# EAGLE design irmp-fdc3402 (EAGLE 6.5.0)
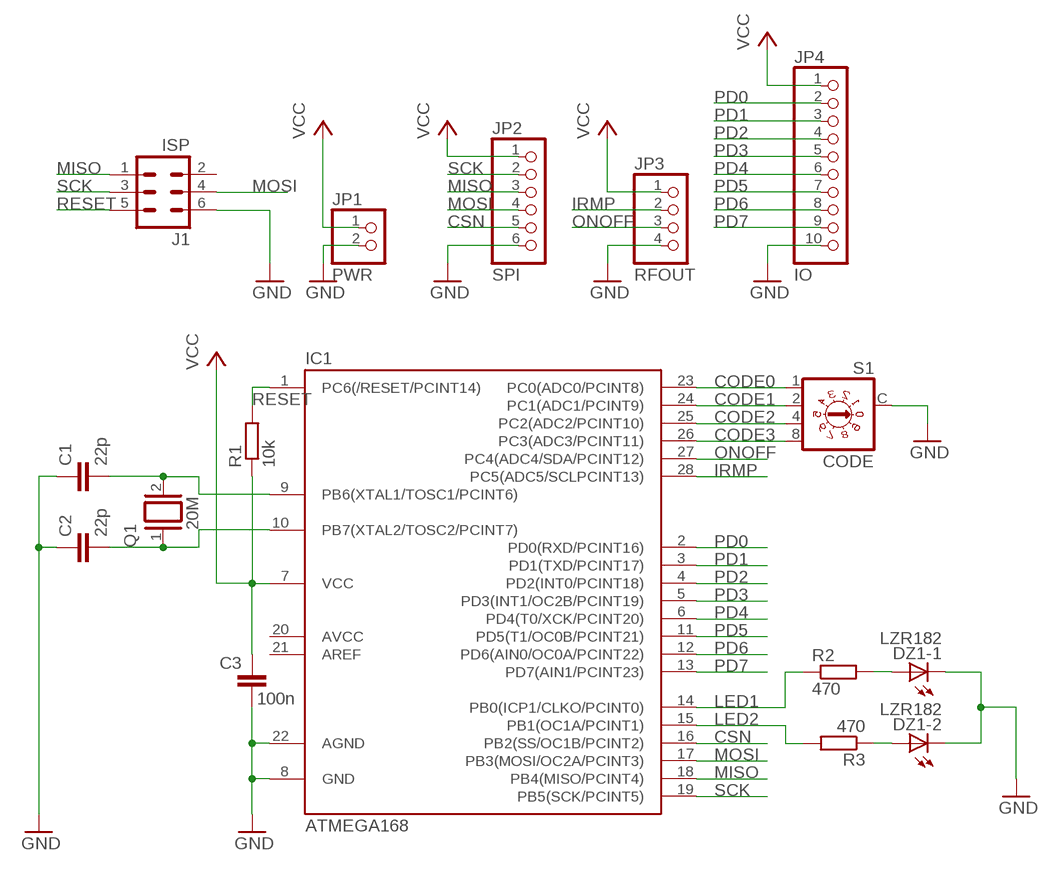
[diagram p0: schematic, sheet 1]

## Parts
C1  22p  C-EU025-024X044  [C025-024X044]
C2  22p  C-EU025-024X044  [C025-024X044]
C3  100n  C-EU025-024X044  [C025-024X044]
DZ1  LZR182  [LZR182]
IC1  ATMEGA168  MEGA48/88/168-PU  [DIL28-3]
J1  ISP  ML6  [ML6]
JP1  PWR  PINHD-1X2  [1X02]
JP2  SPI  PINHD-1X6  [1X06]
JP3  RFOUT  PINHD-1X4  [1X04]
JP4  IO  PINHD-1X10  [1X10]
Q1  20M  XTAL/S  [QS]
R1  10k  R-EU_0207/10  [0207/10]
R2  470  R-EU_0207/10  [0207/10]
R3  470  R-EU_0207/10  [0207/10]
S1  CODE  DRS3010  [DRR3010]

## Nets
CODE0: IC1.23(PC0(ADC0/PCINT8)) S1.1
CODE1: IC1.24(PC1(ADC1/PCINT9)) S1.2
CODE2: IC1.25(PC2(ADC2/PCINT10)) S1.4
CODE3: IC1.26(PC3(ADC3/PCINT11)) S1.8
CSN: IC1.16(PB2(SS/OC1B/PCINT2)) JP2.5
GND: C1.1 C2.1 C3.1 DZ1.K1(-1:C) DZ1.K2(-2:C) IC1.8(GND) IC1.22(AGND) J1.6 JP1.2 JP2.6 JP3.4 JP4.10 S1.C
IRMP: IC1.28(PC5(ADC5/SCLPCINT13)) JP3.2
LED1: IC1.14(PB0(ICP1/CLKO/PCINT0)) R2.1
LED2: IC1.15(PB1(OC1A/PCINT1)) R3.2
MISO: IC1.18(PB4(MISO/PCINT4)) J1.1 JP2.3
MOSI: IC1.17(PB3(MOSI/OC2A/PCINT3)) J1.4 JP2.4
N$1: DZ1.A1(-1:A) R2.2
N$2: DZ1.A2(-2:A) R3.1
ONOFF: IC1.27(PC4(ADC4/SDA/PCINT12)) JP3.3
PD0: IC1.2(PD0(RXD/PCINT16)) JP4.2
PD1: IC1.3(PD1(TXD/PCINT17)) JP4.3
PD2: IC1.4(PD2(INT0/PCINT18)) JP4.4
PD3: IC1.5(PD3(INT1/OC2B/PCINT19)) JP4.5
PD4: IC1.6(PD4(T0/XCK/PCINT20)) JP4.6
PD5: IC1.11(PD5(T1/OC0B/PCINT21)) JP4.7
PD6: IC1.12(PD6(AIN0/OC0A/PCINT22)) JP4.8
PD7: IC1.13(PD7(AIN1/PCINT23)) JP4.9
RESET: IC1.1(PC6(/RESET/PCINT14)) J1.5 R1.2
SCK: IC1.19(PB5(SCK/PCINT5)) J1.3 JP2.2
VCC: C3.2 IC1.7(VCC) JP1.1 JP2.1 JP3.1 JP4.1 R1.1
XTAL1: C1.2 IC1.9(PB6(XTAL1/TOSC1/PCINT6)) Q1.2
XTAL2: C2.2 IC1.10(PB7(XTAL2/TOSC2/PCINT7)) Q1.1
Unconnected: IC1.20(AVCC) IC1.21(AREF) J1.2

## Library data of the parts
C1-C3 = rcl:C-EU: CAPACITOR, European symbol
DZ1 = led:LZR182: LED BLOCK 2 LEDs, Siemens
IC1 = avr-7:MEGA48/88/168-PU
J1 = con-harting-ml:ML6: HARTING; OC_FARNELL: unknown; OC_NEWARK: unknown
JP1 = pinhead:PINHD-1X2: PIN HEADER
JP2 = pinhead:PINHD-1X6: PIN HEADER
JP3 = pinhead:PINHD-1X4: PIN HEADER
JP4 = pinhead:PINHD-1X10: PIN HEADER
Q1 = special:XTAL/S: CRYSTAL
R1-R3 = rcl:R-EU_: RESISTOR, European symbol
S1 = switch-dil:DRS3010: DIL/CODE SWITCH; MPN: DRS3010; OC_FARNELL: 1190426; OC_NEWARK: 01M7366

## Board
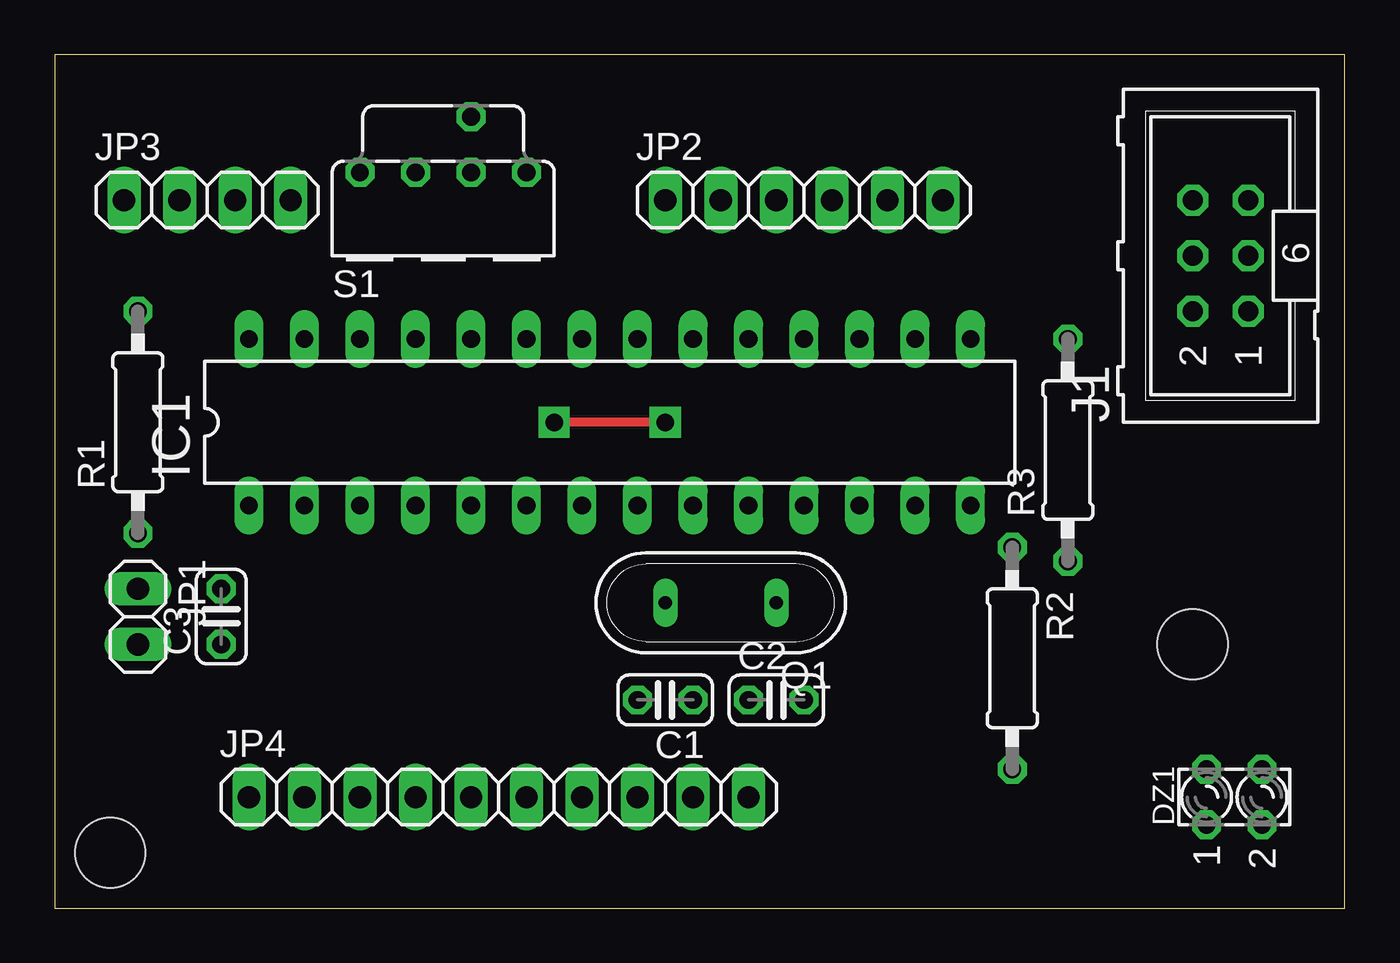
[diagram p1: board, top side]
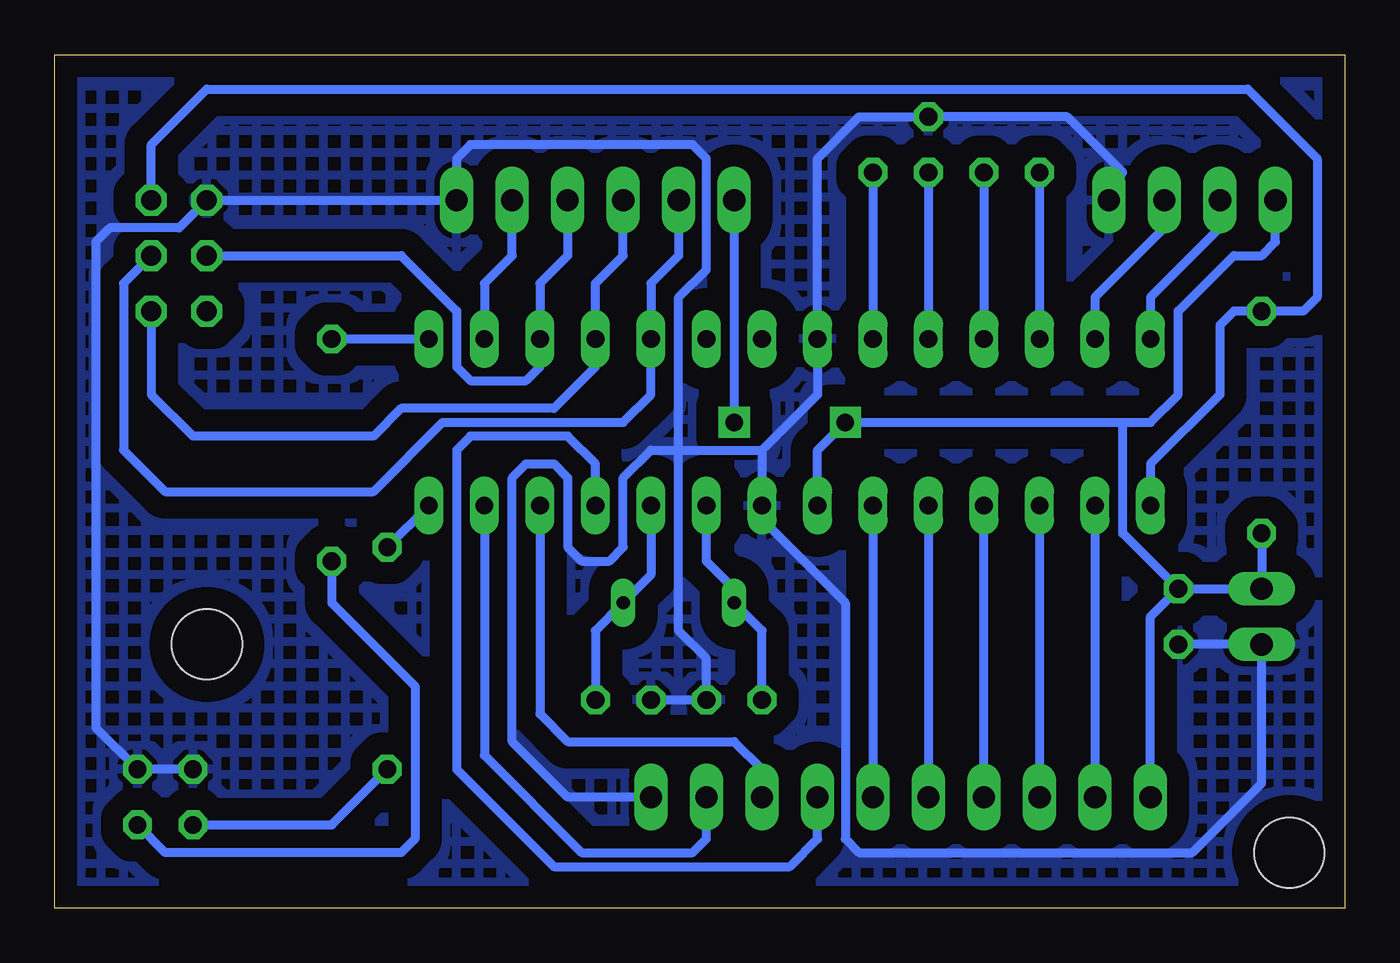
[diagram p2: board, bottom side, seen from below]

Size 59.03 x 39.04 mm. Coordinates in mm from the lower left corner, seen from the top.
Outline: 0,0 59.03,0 59.03,39.04 0,39.04 0,0
Copper layers (1*16): Top 0.035mm / dielectric 1.5mm / Bottom 0.035mm
Design rules "default": minimum track width 10mil, minimum drill 24mil, track to track 8mil, track to pad 8mil, pad to pad 8mil, via to via 8mil, smd to smd 8mil, copper to edge 40mil, drill to drill 8mil, minimum pad ring 10mil, minimum via ring 8mil, stop-mask expansion 4mil, vias tented up to drill 0mil, thermal gap 10mil
Holes 3.2 mm at 2.54,2.54 52.07,12.06

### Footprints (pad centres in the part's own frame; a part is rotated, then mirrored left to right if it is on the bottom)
C025-024X044 = drill 0.813 octagon: 1 -1.27,0; 2 1.27,0
LZR182 = drill 0.813 octagon: A1 -1.27,1.27; A2 -1.27,-1.27; K1 1.27,1.27; K2 1.27,-1.27
DIL28-3 = drill 0.813 long: 1 -16.51,-3.81; 2 -13.97,-3.81; 3 -11.43,-3.81; 4 -8.89,-3.81; 5 -6.35,-3.81; 6 -3.81,-3.81; 7 -1.27,-3.81; 8 1.27,-3.81; 9 3.81,-3.81; 10 6.35,-3.81; 11 8.89,-3.81; 12 11.43,-3.81; 13 13.97,-3.81; 14 16.51,-3.81; 15 16.51,3.81; 16 13.97,3.81; 17 11.43,3.81; 18 8.89,3.81; 19 6.35,3.81; 20 3.81,3.81; 21 1.27,3.81; 22 -1.27,3.81; 23 -3.81,3.81; 24 -6.35,3.81; 25 -8.89,3.81; 26 -11.43,3.81; 27 -13.97,3.81; 28 -16.51,3.81
ML6 = drill 0.914 octagon: 1 -2.54,-1.27; 2 -2.54,1.27; 3 0,-1.27; 4 0,1.27; 5 2.54,-1.27; 6 2.54,1.27
1X02 = drill 1.016 long: 1 -1.27,0; 2 1.27,0
1X06 = drill 1.016 long: 1 -6.35,0; 2 -3.81,0; 3 -1.27,0; 4 1.27,0; 5 3.81,0; 6 6.35,0
1X04 = drill 1.016 long: 1 -3.81,0; 2 -1.27,0; 3 1.27,0; 4 3.81,0
1X10 = drill 1.016 long: 1 -11.43,0; 2 -8.89,0; 3 -6.35,0; 4 -3.81,0; 5 -1.27,0; 6 1.27,0; 7 3.81,0; 8 6.35,0; 9 8.89,0; 10 11.43,0
QS = drill 0.61 long: 1 -2.54,0; 2 2.54,0
0207/10 = drill 0.813 octagon: 1 -5.08,0; 2 5.08,0
DRR3010 = drill 0.813 octagon: 1 3.81,0; 2 1.27,0; 4 -1.27,0; 8 -3.81,0; C 1.27,2.54

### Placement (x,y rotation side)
C1  27.94,9.53 180 top
C2  33.02,9.53 0 top
C3  7.62,13.34 90 top
DZ1  53.98,5.08 90 top
IC1  25.4,22.23 0 top
J1  53.34,29.84 90 top
JP1  3.81,13.34 270 top
JP2  34.29,32.38 0 top
JP3  6.99,32.38 0 top
JP4  20.32,5.08 0 top
Q1  30.48,13.97 180 top
R1  3.81,22.23 90 top
R2  43.81,11.43 270 top
R3  46.35,20.95 90 top
S1  17.78,33.66 0 top

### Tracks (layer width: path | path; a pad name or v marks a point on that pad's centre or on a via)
CODE0
  Bottom 0.406: S1.1 IC1.23
CODE1
  Bottom 0.406: S1.2 IC1.24
CODE2
  Bottom 0.406: S1.4 IC1.25
CODE3
  Bottom 0.406: S1.8 IC1.26
CSN
  Bottom 0.406: IC1.16 39.37,28.57 38.1,29.84 JP2.5
GND
  Bottom 0.406: C3.1 JP1.2 3.81,5.71 6.99,2.54 22.23,2.54 22.86,3.17 22.86,13.97 26.67,17.78 IC1.8 26.67,20.95 | C2.1 C1.1 29.21,11.43 30.48,12.7 30.48,20.95 | 30.48,20.95 26.67,20.95 | 26.67,20.95 24.13,23.5 IC1.22 24.13,34.29 22.23,36.2 S1.C 12.7,36.2 10.16,33.66 JP3.4 | 30.48,20.95 30.48,27.94 29.21,29.21 29.21,34.29 29.84,34.92 40.01,34.92 40.64,34.29 JP2.6 J1.6 53.34,31.11 56.52,31.11 57.15,30.48 57.15,8.26 DZ1.K2 DZ1.K1 | JP4.10 35.56,5.08 38.1,7.62 38.1,19.68 37.47,20.32 36.2,20.32 35.56,19.68 35.56,16.51 34.92,15.88 33.66,15.88 33.02,16.51 33.02,19.68 31.75,20.95 30.48,20.95
  pour Bottom (isolate 1.016, hatched): 0,39.37 59.05,39.37 59.05,0 0,0
IRMP
  Bottom 0.406: JP3.2 5.71,31.11 8.89,27.94 IC1.28
LED1
  Bottom 0.406: IC1.14 R2.1
LED2
  Bottom 0.406: R3.2 IC1.15
MISO
  Bottom 0.406: JP2.3 33.02,29.84 34.29,28.57 IC1.18 34.29,24.77 36.2,22.86 43.18,22.86 44.45,21.59 52.7,21.59 54.61,23.5 J1.1
MOSI
  Bottom 0.406: JP2.4 35.56,29.84 36.83,28.57 IC1.17 36.83,24.77 37.47,24.13 40.01,24.13 40.64,24.77 40.64,27.3 43.18,29.84 J1.4
N$1
  Bottom 0.406: DZ1.A1 46.35,3.81 R2.2
N$2
  Bottom 0.406: R3.1 46.35,13.97 42.55,10.16 42.55,3.17 43.18,2.54 53.98,2.54 DZ1.A2
ONOFF
  Bottom 0.406: JP3.3 8.26,31.11 11.43,27.94 IC1.27
PD0
  Bottom 0.406: IC1.2 JP4.2
PD1
  Bottom 0.406: IC1.3 JP4.3
PD2
  Bottom 0.406: JP4.4 IC1.4
PD3
  Bottom 0.406: IC1.5 JP4.5
PD4
  Bottom 0.406: IC1.6 JP4.6
PD5
  Bottom 0.406: IC1.11 34.29,20.32 35.56,21.59 40.01,21.59 40.64,20.95 40.64,6.35 36.2,1.91 25.4,1.91 24.13,3.17 JP4.7
PD6
  Bottom 0.406: IC1.12 36.83,8.89 35.56,7.62 27.94,7.62 26.67,6.35 JP4.8
PD7
  Bottom 0.406: IC1.13 39.37,6.99 34.92,2.54 29.84,2.54 29.21,3.17 JP4.9
RESET
  Bottom 0.406: IC1.1 8.89,20.32 5.71,23.5 5.71,26.67 5.08,27.3 R1.2 1.91,27.3 1.27,27.94 1.27,34.29 4.45,37.47 52.07,37.47 54.61,34.92 J1.5
SCK
  Bottom 0.406: JP2.2 30.48,29.84 31.75,28.57 IC1.19 31.75,23.5 33.02,22.23 41.27,22.23 44.45,19.05 53.98,19.05 55.88,20.95 55.88,28.57 J1.3
VCC  (via drill 0.8 pad 1.42)
  Top 0.406: v27.94,22.23 v22.86,22.23
  Bottom 0.406: JP3.1 3.17,30.48 3.81,29.84 5.08,29.84 7.62,27.3 7.62,23.5 8.89,22.23 10.16,22.23 | R1.1 JP1.1 C3.2 | JP4.1 8.89,13.34 C3.2 | IC1.7 24.13,20.95 v22.86,22.23 10.16,22.23 | JP2.1 v27.94,22.23 | C3.2 10.16,17.14 10.16,22.23
XTAL1
  Bottom 0.406: IC1.9 29.21,15.88 27.94,14.61 Q1.2 26.67,12.7 C1.2
XTAL2
  Bottom 0.406: IC1.10 31.75,15.24 Q1.1 34.29,12.7 C2.2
